VAR_GLOBAL
	
//	inputs 	AT%IB0 : ARRAY[0..200] OF BYTE;	// define used input space - not used
//	outputs AT%QB0 : ARRAY[0..200] OF BYTE;	// define used output space - not used
	memory 	AT%MB0 : ARRAY[0..200] OF BYTE;	// define used memory space
//	data	: ARRAY[0..200] OF BYTE;		// define used data space - not used


//Datapoints SLAVE -> MASTER (monitoring direction)
	(* Input IW0-99*)	// example

	(* Output QW0-99*)	// example
	
	(* Memory MW0-99*)	// example
		(*Single points*)
		bSlaveToMaster 		AT%MX0.0		: BOOL;	// obj addr: 10 - M_SP_NA_1 at byte/bit offset: 0/0
		
		(*Bitstrings*)
		nBitstring			AT%MD1			: DWORD;	// obj addr: 11 - M_BO_NA_1 at byte offset: 4 (AT%MD1 -> 4*1)		
	
		(*Measurement Value*)
		// scaled value
		nMeasurementValue 	AT%MW10			: INT;	// obj addr: 12 - M_ME_NB_1 at byte offset: 20 (AT%MW10 -> 2*10)
		
		// short floating point value
		fMeasurementValue 	AT%MD6			: REAL;	// obj addr: 13 - M_ME_NC_1 at byte offset: 24 (AT%MD6 -> 4*6)
		
	(* Data *)
	
//Datapoints MASTER -> SLAVE (control directon)
	(* Input IW100-200*)	// example

	(* Output QW100-200*)	// example
	
	(* Memory MW100-200*)	// example
		(*Single commands*)
		bMasterToSlave 		AT%MX100.0		: BOOL;	// obj addr: 101 - C_SC_NA_1 at byte/bit offset: 100/0
		
	(* Data *)
	
//other variables
		
END_VAR
